TYPE ConfigMfcGas :
STRUCT
	Enable:BOOL;
	GasName:STRING;
	N2Scale:SVLREAL;
	ScaleFactor:SVLREAL;
	DefaultSV:SVINT;
	FlowRegulationFactor:SVINT;
	EnableAlarm:BOOL;
	AlarmRange:SVINT;
	AlarmTime:SVINT;
	WarningRange:SVINT;
	WarningTime:SVINT;
	WriteMode:SVINT;
END_STRUCT
END_TYPE
